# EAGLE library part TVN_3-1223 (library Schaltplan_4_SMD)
Isolated DC/DC Converters 3W 9-18Vin SIP-8 +/-15Vout +/-100mA Source: Datasheet
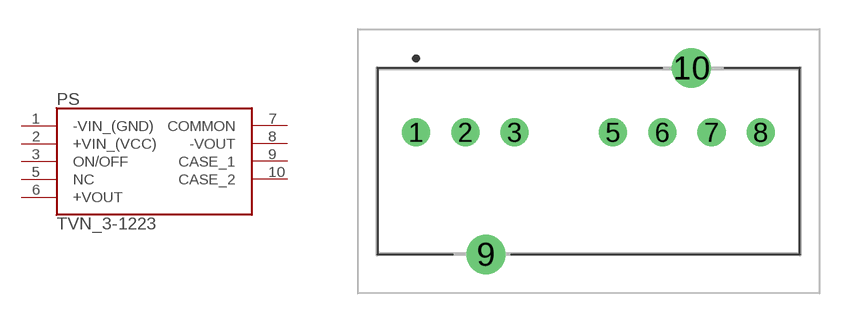
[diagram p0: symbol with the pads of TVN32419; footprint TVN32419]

Designator prefix PS

## TVN_3-1223 (ALLIED_NUMBER: 71099550; ALLIED_PRICE-STOCK: https://www.alliedelec.com/traco-power-tvn-3-1223/71099550/; DESCRIPTION: Isolated DC/DC Converters 3W 9-18Vin SIP-8 +/-15Vout +/-100mA; HEIGHT: 11mm; MANUFACTURER_NAME: Traco Power; MANUFACTURER_PART_NUMBER: TVN 3-1223; MOUSER_PART_NUMBER: 495-TVN3-1223; MOUSER_PRICE-STOCK: https://www.mouser.com/Search/Refine.aspx?Keyword=495-TVN3-1223; RS_PART_NUMBER: 1466094; RS_PRICE-STOCK: https://uk.rs-online.com/web/p/products/1466094)  [TVN32419]
1  -VIN_(GND)
2  +VIN_(VCC)
3  ON/OFF
5  NC  nc
6  +VOUT
7  COMMON
8  -VOUT
9  CASE_1
10  CASE_2

## Footprint TVN32419 (pad centres in mm)
TVN 3 Series
drill 0.89 pad 1.446: 1 -8.9,1.5; 2 -6.36,1.5; 3 -3.82,1.5; 5 1.26,1.5; 6 3.8,1.5; 7 6.34,1.5; 8 8.88,1.5
drill 1.35 pad 2.025: 9 -5.3,-4.8; 10 5.3,4.8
